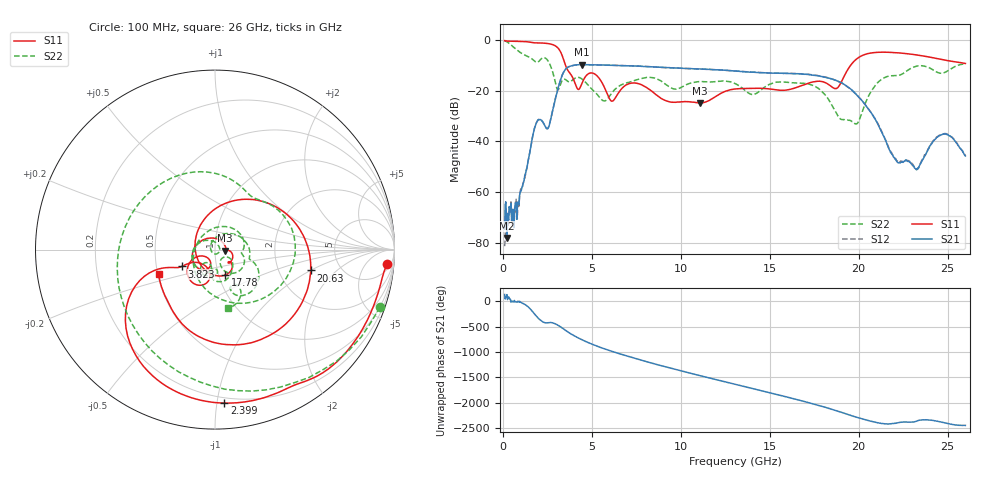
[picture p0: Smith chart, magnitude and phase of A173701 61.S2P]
!  2-Port S-parameters saved by WinCal
! VAR MeasName=S-Parameters (CALIBRATED_DATA) read from VNA (N5245A)
! VAR MeasDate=2017-6-7 10:32:29
! VAR NAME=A173701 61
! VAR FILENAME=A173701 61.S2P
! VAR DATE=2017-6-7 10:32:29
! VAR PHYS_PORTS=1,2
# Hz S DB R 50
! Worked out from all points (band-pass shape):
!   801 points, 100 MHz to 26 GHz, reference 50 ohm
!   highest |S21| = -9.74 dB at 4.438 GHz (marker M1); lowest = -78.1 dB at 229.5 MHz (marker M2)
!   |S21| within 3 dB of the highest: 3.417 GHz to 13.86 GHz (10.45 GHz wide, 121 % of centre)
!   lowest |S11| = -24.9 dB at 11.08 GHz (marker M3), VSWR 1.12, Z = 56 - j0.717 ohm
!   |S11| at or under -10 dB: 3.522 GHz to 19.55 GHz (16.03 GHz wide, 139 % of centre)
!   |S22| runs from -33.2 to -0.2 dB; largest |S21 - S12| = 0.0036
!   S11 on the Smith chart (normalised r, x): 100 MHz: 9, -20; 2.399 GHz: 0.16, -1.05; 3.823 GHz: 0.68, -0.13; 17.78 GHz: 1.07, -0.31; 20.63 GHz: 3.03, -1.00; 26 GHz: 0.51, -0.16
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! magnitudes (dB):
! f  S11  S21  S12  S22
! 100 MHz  -0.3  -74.7  -81.4  -0.2
! 229.5 MHz  -0.5  -78.1  -71.7  -0.7
! 909.4 MHz  -0.6  -64.9  -65.6  -4.6
! 1.881 GHz  -1.2  -32.9  -32.8  -8.8
! 2.399 GHz  -1.3  -34.4  -34.3  -7.2
! 3.079 GHz  -3.1  -19.8  -19.7  -19.7
! 3.823 GHz  -13.6  -10.3  -10.3  -16.4
! 4.438 GHz  -17.3  -9.7  -9.7  -15.4
! 5.021 GHz  -13.1  -9.8  -9.9  -19.6
! 5.701 GHz  -18.6  -10.0  -9.9  -24.1
! 8.744 GHz  -22.3  -10.8  -10.8  -15.7
! 11.08 GHz  -24.9  -11.5  -11.5  -16.5
! 13.05 GHz  -19.4  -12.3  -12.3  -17.2
! 17.39 GHz  -16.6  -13.9  -13.8  -17.9
! 17.78 GHz  -16.3  -14.2  -14.2  -19.4
! 18.78 GHz  -19.1  -16.1  -16.1  -29.3
! 19.82 GHz  -8.0  -21.1  -21.2  -33.2
! 20.63 GHz  -5.3  -28.0  -27.9  -21.2
! 21.69 GHz  -4.9  -42.8  -42.6  -14.3
! 23.28 GHz  -6.0  -51.2  -51.0  -10.3
! 24.87 GHz  -8.0  -37.1  -37.0  -12.8
! 26 GHz  -9.3  -45.8  -45.7  -9.5
